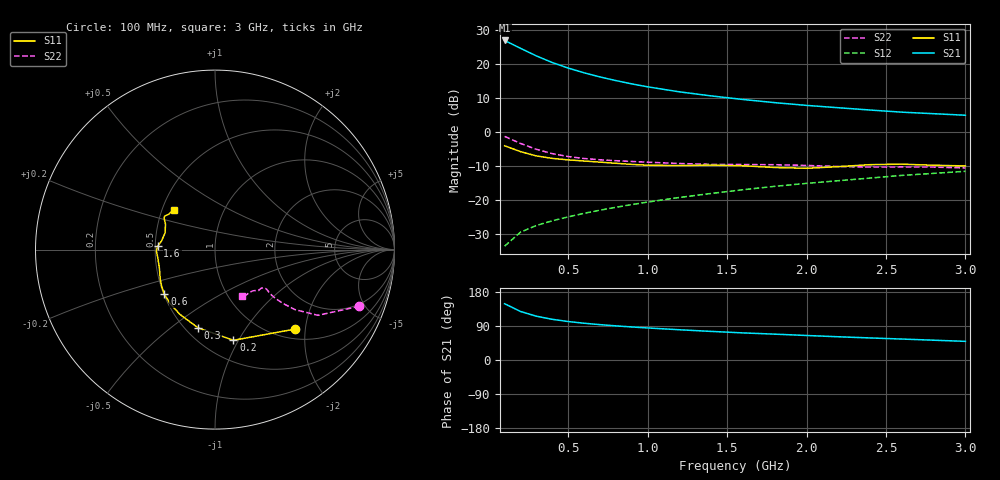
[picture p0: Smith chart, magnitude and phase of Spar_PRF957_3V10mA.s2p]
! Filename:  PRF957E.S2P  Version:  3.0
! NXP part #:  PRF957  Date:  Nov 1998
! Bias condition:  Vce=3V, Ic=10mA
#  MHz  S  MA  R 50
! Freq  S11  S21  S12  S22
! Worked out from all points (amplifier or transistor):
!   20 points, 100 MHz to 3 GHz, reference 50 ohm
!   highest |S21| = 26.9 dB at 100 MHz (marker M1)
!   |S21| within 3 dB of that: start of sweep to 231.1 MHz
!   unconditionally stable (mu >= 1): 1.013 GHz to end of sweep
!   at 400 MHz: K = 0.71, MSG = 23.3 dB, |S12| = -26.1 dB
!   at 1.2 GHz: K = 1.03, MAG = 14.5 dB, |S12| = -19.2 dB
!   at 3 GHz: K = 1.04, MAG = 7.0 dB, |S12| = -11.5 dB
!   S11 on the Smith chart (normalised r, x): 100 MHz: 1.20, -1.76; 200 MHz: 0.69, -0.95; 300 MHz: 0.58, -0.63; 600 MHz: 0.50, -0.29; 1.6 GHz: 0.52, +0.02; 3 GHz: 0.58, +0.29
100  0.629 -44.8  22.16 148.5  0.02106 70.9  0.863 -21.5
200  0.5155 -78.5  16.99 128.1  0.03382 62.4  0.6807 -32.5
300  0.4459 -102.2  13.13 115.5  0.04243 60.2  0.5575 -36.9
400  0.4101 -118.7  10.5 107.4  0.0497 60.8  0.482 -38.4
500  0.39 -130.3  8.708 101.5  0.05674 62.3  0.4365 -38.9
600  0.3754 -138.7  7.422 97.0  0.06393 63.9  0.4087 -38.9
700  0.3614 -145.3  6.451 93.3  0.07114 65.5  0.3913 -38.6
800  0.3476 -151.2  5.705 90.1  0.07845 66.9  0.3794 -38.2
900  0.3347 -156.8  5.1 87.2  0.08594 68.1  0.3697 -37.7
1000  0.3257 -162.3  4.618 84.6  0.09367 69.1  0.361 -37.4
1200  0.3219 -172.2  3.896 79.8  0.1094 70.4  0.3452 -37.9
1400  0.3268 -178.8  3.398 75.5  0.1253 71.1  0.3353 -40.0
1600  0.3197 176.8  3.007 71.5  0.142 71.7  0.3333 -42.1
1800  0.3014 170.6  2.704 68.2  0.1595 71.9  0.3314 -43.4
2000  0.2934 161.2  2.463 64.7  0.1761 72.1  0.3234 -44.7
2200  0.3102 152.7  2.276 61.3  0.1928 72.0  0.3116 -47.5
2400  0.3319 148.6  2.106 58.2  0.2108 71.5  0.3056 -51.5
2600  0.3375 146.5  1.96 55.3  0.2308 70.8  0.3069 -55.1
2800  0.3253 142.8  1.859 52.2  0.2472 70.6  0.3056 -57.3
3000  0.3178 135.4  1.766 49.2  0.2652 70.3  0.297 -59.7
